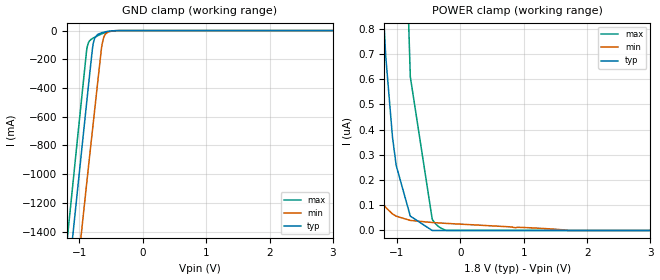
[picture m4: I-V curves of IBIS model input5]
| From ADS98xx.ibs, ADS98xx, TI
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|   input5 Model
[Model]   input5
Model_type   Input
Vinl = 0.54
Vinh = 1.26
|   typ   min   max
C_comp   0.967pF   0.924pF   1.01pF
[Voltage Range]   1.8   1.75   1.85
[Temperature Range]   27   125   -40
[Power Clamp Reference]   1.8   1.75   1.85
[GND Clamp Reference]   0   0   0
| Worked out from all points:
|   GND clamp passes 1 mA (typ) near -0.45 V on its own axis
[GND Clamp]
|   Voltage   I(typ)   I(min)   I(max)
-1.8V     -4.405A    -4.9A      -4.097A
-1.325V   -2.367A    -2.897A    -2.028A
-1.114V   -1.467A    -2.013A    -1.113A
-1.055V   -1.214A    -1.765A    -856.1mA
-1.006V   -1.008A    -1.562A    -646mA
-882mV    -484.2mA   -1.049A    -123.7mA
-784.8mV  -95.4mA    -654mA     -52.46mA
-709.2mV  -26.54mA   -349.8mA   -35.35mA
-649.8mV  -15.31mA   -115.7mA   -23.3mA
-622.8mV  -11.87mA   -56.31mA   -18.45mA
-536.4mV  -4.254mA   -7.165mA   -6.706mA
3.6V      0A         0A         0A
[POWER Clamp]
|   Voltage   I(typ)   I(min)   I(max)
-1.8V     14.36uA    1.444uA    89.59uA
-1.681V   8.615uA    835.3nA    58.79uA
-1.503V   3.781uA    363.2nA    28.77uA
-1.39V    2.154uA    215.7nA    17.29uA
-1.26V    1.089uA    124.1nA    9.234uA
-1.179V   694.6nA    91.6nA     6.08uA
-1.071V   369.6nA    65.5nA     3.399uA
-1.017V   265.5nA    57.23nA    2.495uA
-790.2mV  56.81nA    39.88nA    609.6nA
-444.6mV  0A         31.52nA    44.86nA
-331.2mV  0A         29.76nA    13.28nA
3.6V      0A         0A         0A
